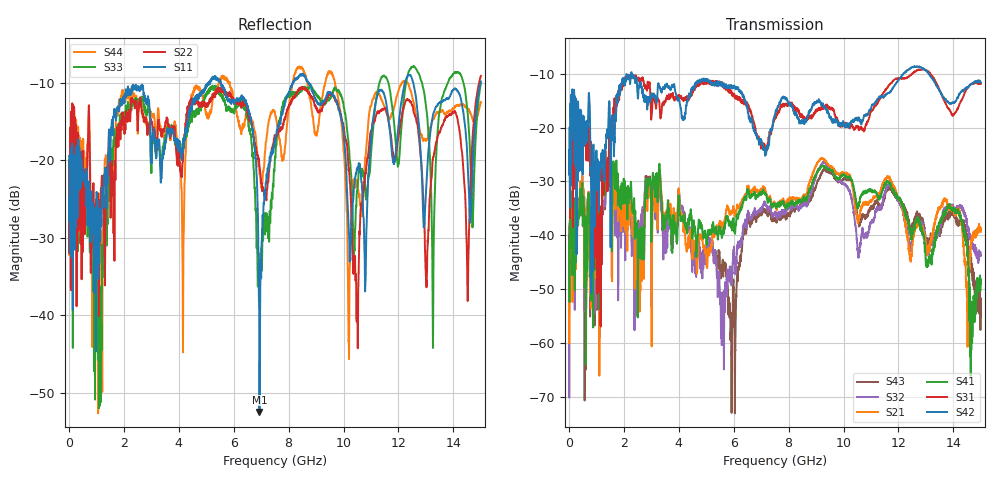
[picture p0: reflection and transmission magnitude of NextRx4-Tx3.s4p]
! FILE: N:\QM 2007\Prüfprotokolle\Highspeed\Konfektionierte Ltg\L45593-D106\D30\8216\0002\Next  Platine 2\NextRx4-Tx3.s4p
# MHz S DB R 50.00
! FREQ  S11  S12  S13  S14
!  S21  S22  S23  S24
!  S31  S32  S33  S34
!  S41  S42  S43  S44
!  DB  ANG  DB  ANG  DB  ANG  DB  ANG
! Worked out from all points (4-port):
!   2999 points, 10 MHz to 15 GHz, reference 50 ohm
!   strongest paths, dB at 10 MHz, 3.755 GHz, 7.505 GHz, 11.26 GHz, 15 GHz:
!     S42: -24.2, -12.0, -17.8, -14.6, -11.6
!     S31: -24.2, -13.8, -18.3, -15.3, -11.8
!     S41: -41.4, -42.4, -34.6, -32.7, -49.0
!     S21: -46.0, -39.5, -34.0, -32.5, -39.3
!     S32: -51.6, -39.2, -35.7, -35.2, -43.7
!     S43: -38.4, -40.1, -37.3, -34.3, -55.2
!   lowest |S11| = -52.4 dB at 6.94 GHz (marker M1), VSWR 1.00, Z = 50 + j0.236 ohm
!   |S11| at or under -10 dB: start of sweep to 5.084 GHz; 5.532 GHz to 8.157 GHz (2.626 GHz wide, 38.4 % of centre); 8.719 GHz to 12.24 GHz (3.522 GHz wide, 33.6 % of centre)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
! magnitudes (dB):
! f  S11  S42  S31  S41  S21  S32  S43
! 10 MHz  -19.4  -24.2  -24.2  -41.4  -46.0  -51.6  -38.4
! 1.465 GHz  -16.4  -15.4  -22.1  -24.8  -25.5  -25.1  -24.5
! 5.365 GHz  -9.7  -11.7  -11.3  -38.4  -39.0  -44.4  -44.6
! 6.94 GHz  -52.4  -22.8  -22.3  -32.2  -32.0  -35.5  -36.1
! 8.255 GHz  -9.7  -17.2  -16.5  -34.0  -33.2  -34.6  -34.8
! 10.49 GHz  -21.0  -18.1  -19.8  -34.5  -37.0  -40.6  -35.7
! 15 GHz  -9.9  -11.6  -11.8  -49.0  -39.3  -43.7  -55.2
